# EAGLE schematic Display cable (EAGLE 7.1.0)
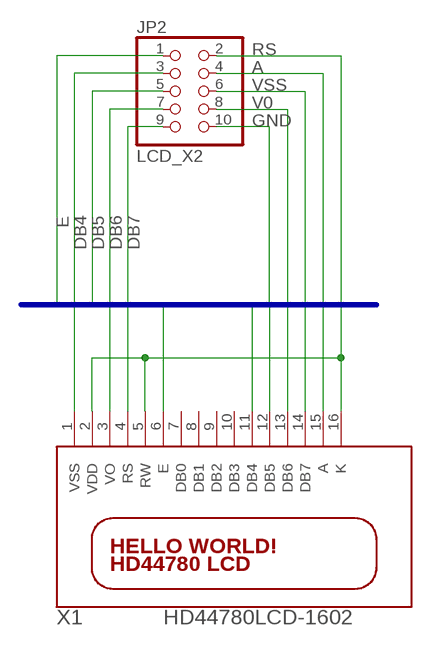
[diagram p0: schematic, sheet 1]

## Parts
JP2  LCD_X2  PINHD-2X5  [2X05]
X1  HD44780LCD-1602  [LCD1602]

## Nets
A: JP2.4 X1.15(A)
DB4: JP2.3 X1.11(DB4)
DB5: JP2.5 X1.12(DB5)
DB6: JP2.7 X1.13(DB6)
DB7: JP2.9 X1.14(DB7)
E: JP2.1 X1.6(E)
GND: JP2.10 X1.2(VDD) X1.5(RW) X1.16(K)
RS: JP2.2 X1.4(RS)
V0: JP2.8 X1.3(VO)
VSS: JP2.6 X1.1(VSS)
Unconnected: X1.7(DB0) X1.8(DB1) X1.9(DB2) X1.10(DB3)

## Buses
VSS,V0,RS,E,DB4,DB5,DB6,DB7,A,GND

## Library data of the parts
JP2 = pinhead:PINHD-2X5: PIN HEADER
X1 = adafruit:HD44780LCD: HD44780 LCD Standard character type LCDs, available in sizes from 8x1 to 40x4!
